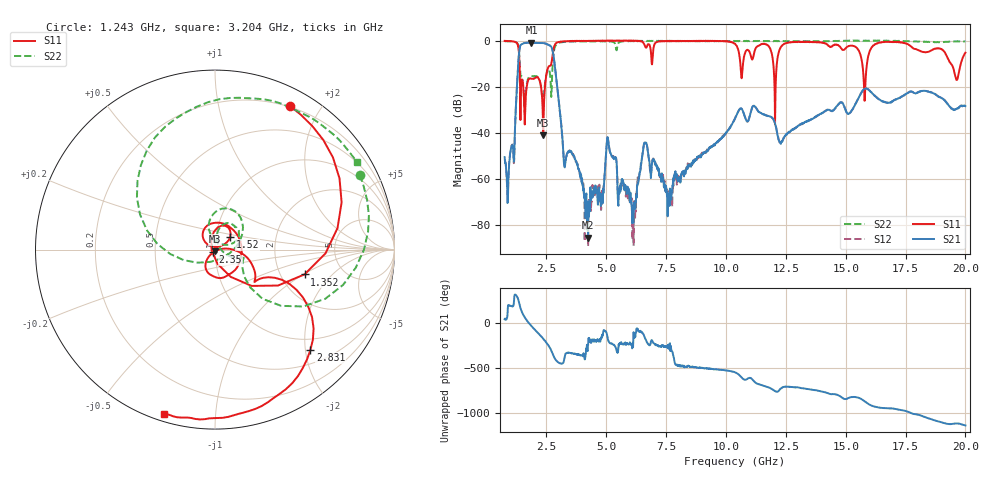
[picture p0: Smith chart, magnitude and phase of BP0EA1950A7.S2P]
! s2p File.  Ports: 1,3
# MHz S DB R 50
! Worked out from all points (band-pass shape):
!   1601 points, 750 MHz to 20 GHz, reference 50 ohm
!   highest |S21| = -0.92 dB at 1.869 GHz (marker M1); lowest = -85.2 dB at 4.239 GHz (marker M2)
!   |S21| within 3 dB of the highest: 1.369 GHz to 2.745 GHz (1.376 GHz wide, 66.9 % of centre)
!   lowest |S11| = -41.1 dB at 2.362 GHz (marker M3), VSWR 1.02, Z = 50.1 - j0.877 ohm
!   |S11| at or under -10 dB: 1.372 GHz to 2.701 GHz (1.329 GHz wide, 65.2 % of centre); 15.69 GHz to 15.89 GHz (196.9 MHz wide, 1.25 % of centre); 19.39 GHz to 19.81 GHz (415.1 MHz wide, 2.12 % of centre)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
!   |S22| runs from -31.2 to 0.0 dB; largest |S21 - S12| = 0.0057
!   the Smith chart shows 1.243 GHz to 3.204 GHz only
!   S11 on the Smith chart (normalised r, x): 1.243 GHz: 0.19, +1.63; 1.352 GHz: 2.71, -1.02; 1.52 GHz: 1.17, +0.17; 2.35 GHz: 0.98, -0.03; 2.831 GHz: 0.76, -2.10; 3.204 GHz: 0.03, -0.74
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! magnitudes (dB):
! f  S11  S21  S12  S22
! 750 MHz  -0.2  -50.4  -51.5  -0.3
! 1.243 GHz  -0.9  -24.1  -24.1  -0.8
! 1.352 GHz  -5.7  -5.6  -5.6  -4.6
! 1.52 GHz  -19.1  -1.3  -1.2  -18.6
! 1.869 GHz  -16.5  -0.9  -0.9  -15.4
! 2.35 GHz  -34.2  -1.1  -1.1  -27.3
! 2.362 GHz  -41.1  -1.1  -1.1  -27.4
! 2.831 GHz  -2.3  -9.5  -9.5  -3.5
! 3.204 GHz  -0.4  -48.6  -48.2  -0.6
! 3.962 GHz  -0.1  -60.8  -59.5  -0.4
! 4.239 GHz  -0.1  -85.2  -89.0  -0.4
! 5.081 GHz  -0.1  -43.4  -43.6  -0.5
! 6.116 GHz  -0.1  -78.5  -74.6  -0.2
! 6.609 GHz  -2.3  -44.4  -44.1  -0.2
! 7.175 GHz  -0.4  -55.8  -56.2  -0.1
! 7.632 GHz  -0.3  -66.7  -68.6  -0.1
! 10.38 GHz  -1.4  -33.7  -33.7  -0.3
! 12.05 GHz  -36.3  -35.8  -35.9  -0.2
! 13.59 GHz  -0.6  -33.8  -33.8  -0.4
! 15.79 GHz  -26.1  -20.8  -20.9  -0.1
! 16.8 GHz  -0.5  -26.8  -26.9  -0.2
! 20 GHz  -5.2  -28.4  -28.4  -0.3
